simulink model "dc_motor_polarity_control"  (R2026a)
settings: Solver=FixedStepAuto  StopTime=inf  EnableMultiTasking=on
libraries: arduinolib x2

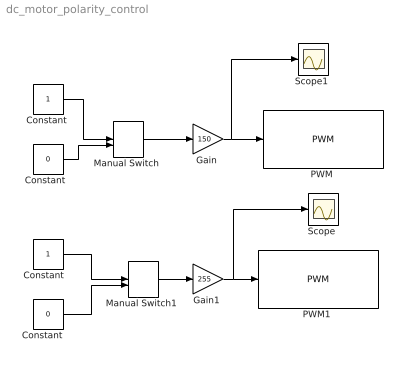
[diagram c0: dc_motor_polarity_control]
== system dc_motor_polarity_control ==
  "Constant " : Constant
  "Constant  " : Constant  Value=0
  "Constant   " : Constant
  "Constant    " : Constant  Value=0
  "Gain " : Gain  Gain=150
  "Gain1 " : Gain  Gain=255
  "Manual Switch " : ManualSwitch
  "Manual Switch1 " : ManualSwitch
  "PWM " : arduinolib/PWM  pinNumber=9  frequencyType=Default  desiredFrequency=490.2  achievableFrequency=490.2
  "PWM1 " : arduinolib/PWM  pinNumber=10  frequencyType=Default  desiredFrequency=490.2  achievableFrequency=490.2
  "Scope " : Scope
  "Scope1 " : Scope
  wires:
  "Constant "/1 -> "Manual Switch "/1
  "Constant  "/1 -> "Manual Switch "/2
  "Constant   "/1 -> "Manual Switch1 "/1
  "Constant    "/1 -> "Manual Switch1 "/2
  "Manual Switch "/1 -> "Gain "/1
  "Gain "/1 -> "Scope1 "/1, "PWM "/1
  "Gain1 "/1 -> "Scope "/1, "PWM1 "/1
  "Manual Switch1 "/1 -> "Gain1 "/1
